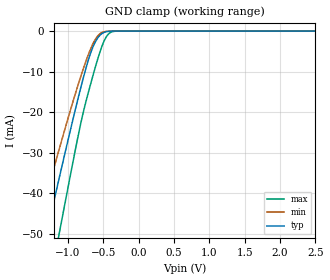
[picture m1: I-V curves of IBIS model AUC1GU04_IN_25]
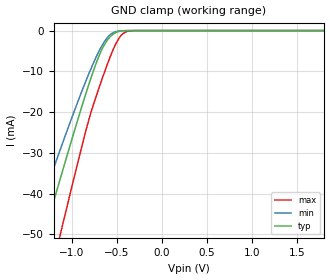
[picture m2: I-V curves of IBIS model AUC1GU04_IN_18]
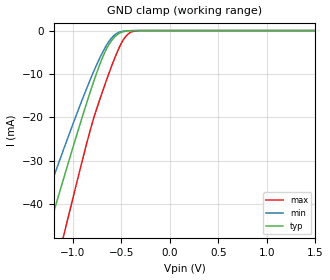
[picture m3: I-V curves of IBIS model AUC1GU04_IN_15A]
| TEXAS INSTRUMENTS INCORPORATED
| Standard Linear and Logic Group
| IBIS Model of SN74AUC1GU04
| Single Gate Inverter
| This file contains package information for the following:
|  SOT 5-pin (DCK) package as [Component] AUC1GU04_DCK
|  SOT 5-pin (DBV) package as [Component] AUC1GU04_DBV
|  NanoStar WCSP 5-pin (YEA) package as [Component] AUC1GU04_YEA
|  NanoFree WCSP 5-pin (YZA) package as [Component] AUC1GU04_YZA
|  NanoStar WCSP 5-pin (YEP) package as [Component] AUC1GU04_YEP
|  NanoFree WCSP 5-pin (YZP) package as [Component] AUC1GU04_YZP
| This device can be powered at the following Vccs:
|  2.5 volt Vcc
|  1.8 volt Vcc
|  1.5 volt Vcc
|  1.2 volt Vcc
|  0.8 volt Vcc
| This file provides unique models under the [Model Selector] for each Vcc.
| For operation at a specific Vcc, select the appropriate model after each
| [Model Selector] keyword.
[IBIS Ver]   3.2
[Comment char]  |_char
[File Name]   sn74auc1gu04.ibs
[File Rev]   1.2 | a_die
[Date]   October 15, 2003
[Source]   Data created from TI-SPICE simulations at TI-SLL.
[Notes]   The following is an IBIS list for the AUC1GU04.
   Please contact sllibis@ti.com with questions and
   comments concerning SLL IBIS models.
[Disclaimer] Property of Texas Instruments Incorporated.  Unauthorized
   reproduction and/or distribution is strictly prohibited.
   This product is protected under copyright law.
   Created  2002, (C) Copyright  2002, Texas Instruments
   Incorporated, All Rights Reserved
   UNLESS THERE IS A SIGNED, WRITTEN AGREEMENT TO THE
   CONTRARY, TEXAS INSTRUMENTS (TI) IS PROVIDING THE IBIS
   MODELS  AND WITHOUT ANY WARRANTY, EXPRESSED OR
   IMPLIED.  TI assumes no liability for:
   1) the accuracy of the IBIS models provided to your
   company;
   2) the proper functioning of these IBIS Models in your
   design or for any resulting applications; or
   3) infringement of patents, copyrights or intellectual
   property rights resulting from your use of these IBIS
   models.
   TI provides IBIS Models as a service to our customers.
   You and your company shall not distribute, sell or give
   these models to anyone else without prior written
   permission from TI.
   TI reserves the right to make changes to our products or
   to discontinue any semiconductor product or service
   without notice, and advises our customers to obtain the
   latest version of relevant information to verify, before
   placing orders, that the information being relied on is
   current.
   Please be aware that your receipt and use of the IBIS
   information provided shall serve as acceptance of these
   terms and conditions.  If you do not accept these terms,
   you should return or destroy the IBIS models and any
   other accompanying information immediately.
| Component AUC1GU04_DCK 5-pin SOT
[Component]   AUC1GU04_DCK
[Manufacturer]   Texas Instruments, Inc.
[Package]
|   typ   min   max
R_pkg   2.000e-02   1.700e-02   2.500e-02
L_pkg   9.980e-10   8.810e-10   1.069e-09
C_pkg   1.460e-13   1.180e-13   2.050e-13
[Pin]   signal_name   model_name   R_pin   L_pin   C_pin
1   NC   NC   1.900e-02   1.069e-09   1.620e-13
2   A   AUC1GU04_IN   1.800e-02   8.810e-10   1.210e-13
3   GND   GND   1.700e-02   1.031e-09   2.050e-13
4   Y   AUC1GU04_OUT   2.000e-02   9.600e-10   1.240e-13
5   VCC   POWER   2.500e-02   1.049e-09   1.180e-13
| Component AUC1GU04_DBV 5-pin SOT
[Component]   AUC1GU04_DBV
[Manufacturer]   Texas Instruments, Inc.
[Package]
|   typ   min   max
R_pkg   2.500e-02   2.100e-02   2.900e-02
L_pkg   1.529e-09   1.312e-09   1.906e-09
C_pkg   1.560e-13   1.100e-13   2.400e-13
[Pin]   signal_name   model_name   R_pin   L_pin   C_pin
1   NC   NC   2.100e-02   1.511e-09   1.440e-13
2   A   AUC1GU04_IN   2.300e-02   1.312e-09   1.380e-13
3   GND   GND   2.900e-02   1.906e-09   2.400e-13
4   Y   AUC1GU04_OUT   2.600e-02   1.541e-09   1.500e-13
5   VCC   POWER   2.500e-02   1.374e-09   1.100e-13
| Component AUC1GU04_YEA 5-pin NanoStar WCSP
[Component]   AUC1GU04_YEA
[Manufacturer]   Texas Instruments, Inc.
[Package]
|   typ   min   max
R_pkg   0.001   0.001   0.001
L_pkg   0.021nH   0.021nH   0.021nH
C_pkg   0.046pF   0.045pF   0.047pF
[Pin]   signal_name   model_name   R_pin   L_pin   C_pin
1   DNU   NC   0.001   0.021nH   0.046pF
2   A   AUC1GU04_IN   0.001   0.021nH   0.047pF
3   GND   GND   0.001   0.021nH   0.046pF
4   Y   AUC1GU04_OUT   0.001   0.021nH   0.045pF
5   VCC   POWER   0.001   0.021nH   0.045pF
| Component AUC1GU04_YZA 5-pin NanoFree WCSP
[Component]   AUC1GU04_YZA
[Manufacturer]   Texas Instruments, Inc.
[Package]
|   typ   min   max
R_pkg   0.001   0.001   0.001
L_pkg   0.021nH   0.021nH   0.021nH
C_pkg   0.046pF   0.045pF   0.047pF
[Pin]   signal_name   model_name   R_pin   L_pin   C_pin
1   DNU   NC   0.001   0.021nH   0.046pF
2   A   AUC1GU04_IN   0.001   0.021nH   0.047pF
3   GND   GND   0.001   0.021nH   0.046pF
4   Y   AUC1GU04_OUT   0.001   0.021nH   0.045pF
5   VCC   POWER   0.001   0.021nH   0.045pF
| Component AUC1GU04_YEP 5-pin NanoStar WCSP
[Component]   AUC1GU04_YEP
[Manufacturer]   Texas Instruments, Inc.
[Package]
|   typ   min   max
R_pkg   0.001   0.001   0.001
L_pkg   0.021nH   0.021nH   0.021nH
C_pkg   0.046pF   0.045pF   0.047pF
[Pin]   signal_name   model_name   R_pin   L_pin   C_pin
1   DNU   NC   0.001   0.021nH   0.046pF
2   A   AUC1GU04_IN   0.001   0.021nH   0.047pF
3   GND   GND   0.001   0.021nH   0.046pF
4   Y   AUC1GU04_OUT   0.001   0.021nH   0.045pF
5   VCC   POWER   0.001   0.021nH   0.045pF
| Component AUC1GU04_YZP 5-pin NanoFree WCSP
[Component]   AUC1GU04_YZP
[Manufacturer]   Texas Instruments, Inc.
[Package]
|   typ   min   max
R_pkg   0.001   0.001   0.001
L_pkg   0.021nH   0.021nH   0.021nH
C_pkg   0.046pF   0.045pF   0.047pF
[Pin]   signal_name   model_name   R_pin   L_pin   C_pin
1   DNU   NC   0.001   0.021nH   0.046pF
2   A   AUC1GU04_IN   0.001   0.021nH   0.047pF
3   GND   GND   0.001   0.021nH   0.046pF
4   Y   AUC1GU04_OUT   0.001   0.021nH   0.045pF
5   VCC   POWER   0.001   0.021nH   0.045pF
| Model AUC1GU04_IN
[Model Selector]   AUC1GU04_IN
AUC1GU04_IN_25   2.5 volt Vcc
AUC1GU04_IN_18   1.8 volt Vcc
AUC1GU04_IN_15A   1.5 volt Vcc
AUC1GU04_IN_12   1.2 volt Vcc
AUC1GU04_IN_08   0.8 volt Vcc
| Model AUC1GU04_OUT
[Model Selector]   AUC1GU04_OUT
AUC1GU04_OUT_25   2.5 volt Vcc
AUC1GU04_OUT_18   1.8 volt Vcc
AUC1GU04_OUT_15A   1.5 volt Vcc
AUC1GU04_OUT_12   1.2 volt Vcc
AUC1GU04_OUT_08   0.8 volt Vcc
| Models and submodels in the file (10): AUC1GU04_IN_25 (Input), AUC1GU04_IN_18 (Input), AUC1GU04_IN_15A (Input), AUC1GU04_IN_12 (Input), AUC1GU04_IN_08 (Input), AUC1GU04_OUT_25 (Output), AUC1GU04_OUT_18 (Output), AUC1GU04_OUT_15A (Output), AUC1GU04_OUT_12 (Output), AUC1GU04_OUT_08 (Output)
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[Model]   AUC1GU04_IN_25
Model_type  Input
Vinl=0.7
Vinh=1.7
| variable   typ   min   max
C_comp   2.66pF   2.24pF   3.22pF
[Temperature Range]   40   100   -40
| Ambient temperature   25   85   -40
[Voltage range]   2.5   2.3   2.7
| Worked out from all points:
|   GND clamp passes 1 mA (typ) near -0.55 V on its own axis
[GND Clamp]
| AUC1GU04_IN_25
|   Voltage   I(typ)   I(min)   I(max)
-3.6V     -230.2mA   -193.8mA   -275.4mA
-1.465V   -62.46mA   -50.68mA   -81.32mA
-1.41V    -58.19mA   -47.14mA   -76.26mA
-1.3V     -49.69mA   -40.13mA   -66.14mA
-1.11V    -35.19mA   -28.25mA   -48.67mA
-845mV    -15.76mA   -12.61mA   -24.92mA
-720mV    -7.623mA   -6.181mA   -15.69mA
-625mV    -3.09mA    -2.403mA   -9.633mA
-515mV    -559.5uA   -308.9uA   -3.552mA
-430mV    -73.2uA    -35.77uA   -776.9uA
-325mV    -3.339uA   -2.035uA   -30.74uA
2.5V      313.9pA    402pA      470.4pA
[Model]   AUC1GU04_IN_18
Model_type  Input
Vinl=0.5775
Vinh=1.2675
| variable   typ   min   max
C_comp   2.64pF   2.26pF   3.19pF
[Temperature Range]   40   100   -40
| Ambient temperature   25   85   -40
[Voltage range]   1.8   1.65   1.95
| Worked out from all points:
|   GND clamp passes 1 mA (typ) near -0.55 V on its own axis
[GND Clamp]
| AUC1GU04_IN_18
|   Voltage   I(typ)   I(min)   I(max)
-3.6V     -230.2mA   -193.8mA   -275.4mA
-1.445V   -60.91mA   -49.39mA   -79.48mA
-1.29V    -48.93mA   -39.5mA    -65.22mA
-1.145V   -37.84mA   -30.41mA   -51.89mA
-1.1V     -34.44mA   -27.64mA   -47.76mA
-830mV    -14.72mA   -11.79mA   -23.67mA
-690mV    -5.96mA    -4.844mA   -13.74mA
-565mV    -1.381mA   -914.2uA   -6.102mA
-490mV    -326uA     -167.9uA   -2.495mA
-425mV    -63.97uA   -31.34uA   -688.8uA
-275mV    -662.6nA   -487.6nA   -4.372uA
1.8V      203.2pA    298.4pA    235.5pA
[Model]   AUC1GU04_IN_15A
Model_type  Input
Vinl=0.49
Vinh=1.04
| variable   typ   min   max
C_comp   2.64pF   2.26pF   3.17pF
[Temperature Range]   40   100   -40
| Ambient temperature   25   85   -40
[Voltage range]   1.5   1.4   1.6
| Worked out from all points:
|   GND clamp passes 1 mA (typ) near -0.55 V on its own axis
[GND Clamp]
| AUC1GU04_IN_15A
|   Voltage   I(typ)   I(min)   I(max)
-3.6V     -230.2mA   -193.8mA   -275.4mA
-1.39V    -56.64mA   -45.86mA   -74.42mA
-1.25V    -45.85mA   -36.97mA   -61.54mA
-1.095V   -34.06mA   -27.33mA   -47.3mA
-1.05V    -30.68mA   -24.59mA   -43.18mA
-810mV    -13.36mA   -10.7mA    -22.06mA
-685mV    -5.701mA   -4.633mA   -13.41mA
-565mV    -1.381mA   -914.2uA   -6.102mA
-490mV    -326uA     -167.9uA   -2.495mA
-425mV    -63.97uA   -31.34uA   -688.8uA
-280mV    -781.4nA   -563.5nA   -5.358uA
1.5V      165.9pA    259.7pA    172.1pA
